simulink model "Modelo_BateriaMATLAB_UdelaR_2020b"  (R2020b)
settings: Solver=VariableStepAuto  StartTime=0.0  StopTime=inf  RelTol=1e-3
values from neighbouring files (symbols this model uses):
  Ic = Q*5/Q    (= 5)    [Parametros_A123.m]    (also in Parametros_A123_pack.m = 69)
  Id = Q*3/Q    (= 3)    [Parametros_A123.m]    (also in Parametros_A123_pack.m = 69)
  Umin = 2    [Parametros_A123.m]    (also in Parametros_A123_pack.m = 400)
undefined symbols (not defined in the file or in its folder): Ion, LiFePO4, Lithium
libraries: powerlib x2, electricdrivelib x1, simulink x1, dspswit3 x1

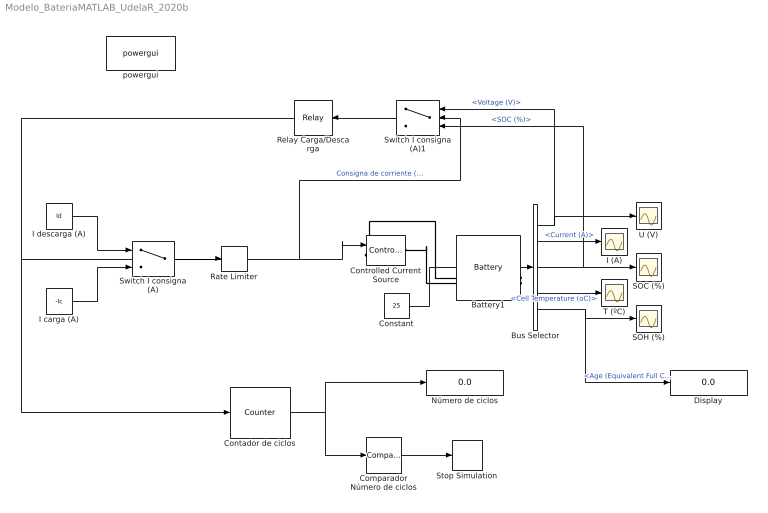
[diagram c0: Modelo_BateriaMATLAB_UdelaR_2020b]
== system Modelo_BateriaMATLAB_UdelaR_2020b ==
  Battery1 : electricdrivelib/Extra Sources/Battery  BatType=Lithium-Ion  ShowTempParam=on  ThermalPreset="3.3V  2.3Ah  (LiFePO4)"  ShowAgeParam=on  NomV=3.3  NomQ=2.3  SOC=100  Batt_Tr=30  PresetModel=off  MaxQ=2.3  MinV=2.475  FullV=3.748  Dis_rate=2.3  R=0.014  Normal_OP=2.25  expZone="[3.4788       0.113]"  current=[6.5 13 32.5]  Units=Time  Tci=20  NomT=25  T2=0  MaxQ2=2.208  FullV2=3.45  Normal_OP2=2.85  expZone2="[3.22       0.015]"  Rca=0.6  ti=1000  Dp=0  Neq0=0  Tsim=1  Ta1=25  Qeol=2.3*0.8  Reol=0.013333*1.2  Char_age=[2.3478, 3]  Dis_age=[2.3478, 10]  N1=1500  N2=10500  N3=1000  N4=1400  Ta2=45  N5=950
  Bus Selector : BusSelector  OutputSignals=Voltage (V),Current (A),SOC (%),Cell Temperature (oC),Age (Equivalent Full Cycles)
  Comparador Número de ciclos : simulink/Logic and Bit Operations/Compare To Constant  relop=>=  const=500  OutDataTypeStr=boolean
  Constant : Constant  Value=25
  Contador de ciclos : dspswit3/Counter  Direction=Up  CountEvent=Either edge  CounterSize=User defined  MaxCount=10000  InitialCount=0  Output=Count  HitValue=32  ResetInput=off  SamplesPerFrame=1  Ts=1  CntDtype=double  HitDtype=Logical
  Controlled Current Source : powerlib/Electrical Sources/Controlled Current Source  Initialize=on  Source_Type=AC  Amplitude=0  Phase=0  Frequency=0  Measurements=None
  Display : Display
  I (A) : Scope
  I carga (A) : Constant  Value=-Ic
  I descarga (A) : Constant  Value=Id
  Número de ciclos : Display
  Rate Limiter : RateLimiter  RisingSlewLimit=inf  FallingSlewLimit=-inf  SampleTimeMode=inherited
  Relay Carga/Descarga : Relay  OnSwitchValue=100  OffSwitchValue=Umin
  SOC (%) : Scope
  SOH (%) : Scope
  Stop Simulation : Stop
  Switch I consigna (A) : Switch  Criteria=u2 > Threshold  Threshold=0.5
  Switch I consigna (A)1 : Switch  Criteria=u2 > Threshold
  T (ºC) : Scope
  U (V) : Scope
  powergui : powerlib/powergui  Priority=1  SimulationMode=Continuous  SampleTime=50e-6  frequency=60  Iterations=50  frequencyindice=0  Pbase=100e6  ErrMax=1e-4  UnitsV=kV  UnitsW=MW  buscounter=0  FunctionMessages=off  echomessages=off  EnableUseOfTLC=off  CurrentSourceSwitches=off  DisableSnubberDevices=off  DisableRonSwitches=off  DisableVfSwitches=off  DisplayEquations=off  AutomaticDiscreteSolvers=off  SolverType=Tustin/Backward Euler (TBE)  Interpol=off  ExternalGateDelay=off  methode=off  Ts=100  x0status=blocks  SPID=on  SwTol=0  HookPort=off  NonlinearTolerance=1e-4  nMaxIteration=100  ContinueOnMaxIteration=off  RestoreLinks=warning  ResistiveCurrentMeasurement=off  Frange=[0:2:500]  Ylog=off  Xlog=on  ShowGrid=off  save=off  variable=ZData  structure=0  ZoomFFT=off  StartTime=0.0  cycles=1  DisplayStyle=1  fundamental=60  FreqAxis=off  MaxFrequency=1000  frequencyindicesteady=1  RmsSteady=1  display=off
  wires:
  Relay Carga/Descarga/1 -> Switch I consigna (A)/2, Contador de ciclos/1
  I descarga (A)/1 -> Switch I consigna (A)/1
  I carga (A)/1 -> Switch I consigna (A)/3
  Switch I consigna (A)/1 -> Rate Limiter/1
  Switch I consigna (A)1/1 -> Relay Carga/Descarga/1
  Battery1/1 -> Bus Selector/1
  Bus Selector/1 -> Switch I consigna (A)1/1, U (V)/1  "<Voltage (V)>"
  Bus Selector/2 -> I (A)/1  "<Current (A)>"
  Bus Selector/3 -> Switch I consigna (A)1/3, SOC (%)/1  "<SOC (%)>"
  Bus Selector/4 -> T (ºC)/1  "<Cell Temperature (oC)>"
  Bus Selector/5 -> Display/1, SOH (%)/1  "<Age (Equivalent Full Cycles)>"
  Constant/1 -> Battery1/1
  Comparador Número de ciclos/1 -> Stop Simulation/1
  Contador de ciclos/1 -> Número de ciclos/1, Comparador Número de ciclos/1
  Rate Limiter/1 -> Controlled Current Source/1, Switch I consigna (A)1/2  "Consigna de corriente (A)"
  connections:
  Controlled Current Source/RConn1 -- Battery1/LConn2
  Controlled Current Source/LConn1 -- Battery1/LConn1
